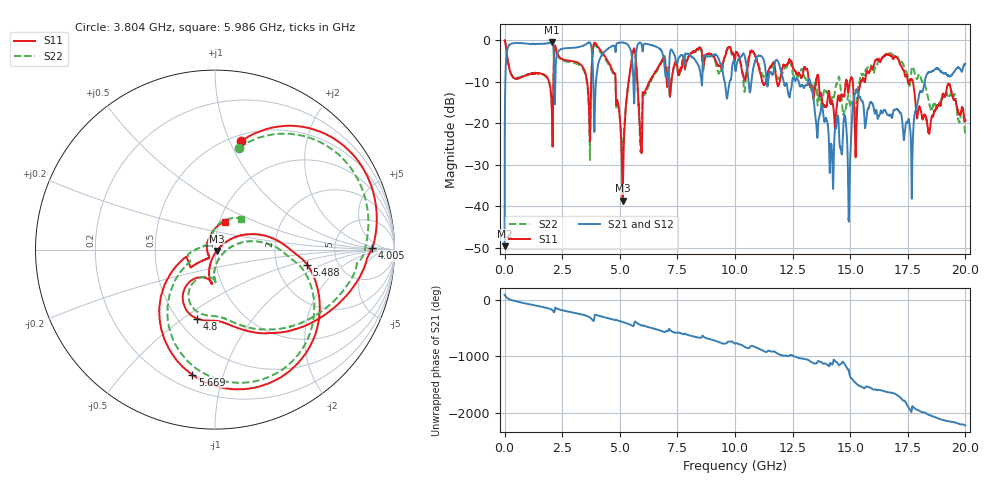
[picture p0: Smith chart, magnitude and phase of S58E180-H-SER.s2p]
!{S58E180}
!Johanson Technology Inc.
!www.johansontechnology.com
!Test Board Conditions:
!Substrate Type  RO4350B
!Substrate Thickness  60 mil
!Substrate Dk  3.66
!TL Type: GCPW
!TL Trace Width  115 mil
!TL Gap  52 mil
!Electrode orientation  Horizontal
!DUT TOPOLOGY	SERIES
!Mounting Pad LxW  55x428 mil
! Created Wed Apr 14 11:21:18 2021
# mhz S ma R 50
! 2 Port Network Data from SP1.SP block
! freq  magS11  angS11  magS21  angS21  magS12  angS12  magS22  angS22
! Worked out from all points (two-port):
!   20001 points, 300 kHz to 20 GHz, reference 50 ohm
!   highest |S21| = -0.47 dB at 2.038 GHz (marker M1); lowest = -49.6 dB at 300 kHz (marker M2)
!   |S21| within 3 dB of the highest: 84.25 MHz to 2.132 GHz (2.047 GHz wide, 185 % of centre); 2.272 GHz to 3.8 GHz (1.528 GHz wide, 50.3 % of centre)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
!   lowest |S11| = -38.6 dB at 5.12 GHz (marker M3), VSWR 1.02, Z = 50.9 - j0.804 ohm
!   |S11| at or under -10 dB: 4.82 GHz to 5.379 GHz (559.1 MHz wide, 11 % of centre); 13.64 GHz to 14.81 GHz (1.169 GHz wide, 8.22 % of centre); 17.72 GHz to end of sweep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
!   |S22| runs from -28.8 to 0.0 dB; largest |S21 - S12| = 0.013
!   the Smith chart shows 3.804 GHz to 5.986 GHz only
!   S11 on the Smith chart (normalised r, x): 3.804 GHz: 0.56, +1.10; 4.005 GHz: 15, +1; 4.8 GHz: 0.62, -0.57; 5.488 GHz: 2.99, -0.69; 5.669 GHz: 0.28, -0.79; 5.986 GHz: 1.06, +0.34
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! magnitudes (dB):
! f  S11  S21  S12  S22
! 300 kHz  0.0  -49.6  -49.5  0.0
! 182.3 MHz  -6.2  -1.2  -1.2  -6.1
! 2.038 GHz  -14.9  -0.5  -0.5  -14.9
! 2.239 GHz  -2.2  -4.6  -4.6  -2.5
! 3.334 GHz  -6.0  -1.4  -1.4  -6.4
! 3.804 GHz  -4.2  -3.8  -3.8  -4.7
! 4.005 GHz  -1.1  -7.8  -7.8  -1.6
! 4.8 GHz  -8.0  -2.0  -2.0  -8.8
! 5.12 GHz  -38.6  -0.5  -0.5  -26.5
! 5.488 GHz  -5.7  -2.6  -2.6  -6.0
! 5.669 GHz  -3.0  -6.7  -6.7  -3.4
! 5.986 GHz  -15.7  -2.6  -2.6  -13.0
! 6.667 GHz  -6.4  -1.8  -1.8  -6.8
! 10 GHz  -4.6  -6.5  -6.5  -4.2
! 13.33 GHz  -10.8  -11.6  -11.6  -12.0
! 14.78 GHz  -11.5  -18.2  -18.1  -16.9
! 14.95 GHz  -11.4  -43.1  -42.6  -14.2
! 15.25 GHz  -26.8  -12.1  -12.1  -17.6
! 16.67 GHz  -3.5  -18.0  -17.8  -3.1
! 17.67 GHz  -9.4  -35.0  -35.4  -6.9
! 18.36 GHz  -20.7  -7.9  -7.8  -13.2
! 20 GHz  -19.3  -5.6  -5.5  -22.3
